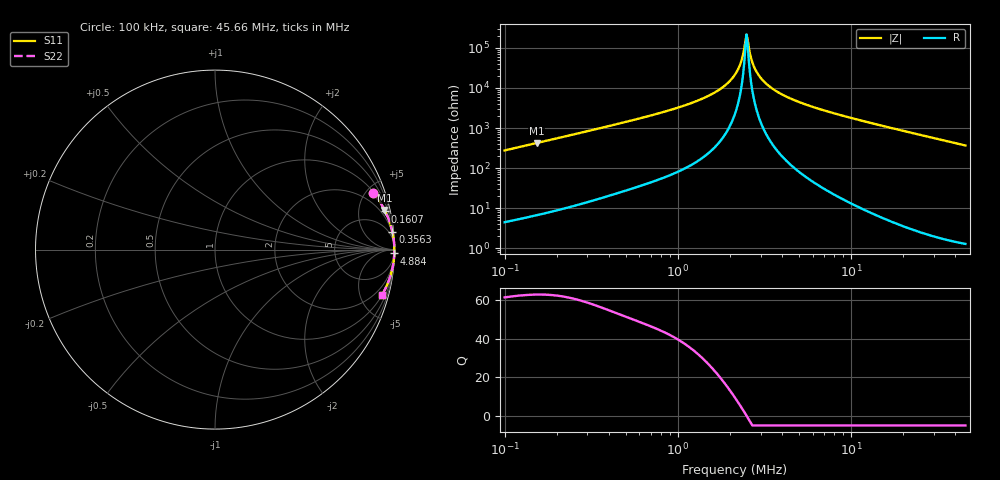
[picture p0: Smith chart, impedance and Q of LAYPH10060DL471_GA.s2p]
! LAYPH10060DL471_GA  S-PARAMETER MODEL  ( General Type )
! Model Generated by TAIYO YUDEN Corporation (http://www.ty-top.com)
! Version 3.0
! TAIYO YUDEN Control No. 180828NI43SB-FBB
! Copyright(c) 2017 TAIYO YUDEN CO.,LTD. All Rights Reserved.
! Product Description (link to TY-COMPAS)
! https://ds.yuden.co.jp/TYCOMPAS/or/detail?pn=LAYPH10060DL471MGA&u=M
! Products Name : Inductors
! Characteristics :
!  Inductance : 470 uH , SRF(min) : -Hz , DC Resistance(max) : 0.93 Ohm
!  Rated Current : Saturation :0.65 A , Temp Rise : 0.39 A (25 degC)
!  Case Size : 10.1 x 10.0 / 0.398 x 0.394 [mm/inch] , Thickness : 6 / 0.236 [mm/inch]
!  (Conditions: Temperature = 25 degC , DC Bias Current/Voltage = 0A / 0V)
! External Node Assignments :
!  1  o---GGG---o  2
! GND o---------o GND
! Frequency Range : 0.1MHz  -  45.660989MHz  [ 402 STEP ]
# MHz S RI R 50
! Freq[MHz].  S11 Real  S11 Imag  S21 Real  S21 Imag  S12 Real  S12 Imag  S22 Real  S22 Imag
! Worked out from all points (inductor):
!   401 points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, 100 kHz to 45.66 MHz, reference 50 ohm
!   read as one part in series: L = 439 uH near 103.1 kHz
!   highest Q = 63 at 153.5 kHz (marker M1), where L = 440 uH
!   self-resonance near 2.49 MHz
!   S11 on the Smith chart (normalised r, x): 100 kHz: 1.09, +5.54; 160.7 kHz: 1.14, +8.89; 356.3 kHz: 1, +20; 4.884 MHz: 3, -93; 45.66 MHz: 1.03, -7.37
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0.1  0.8808 0.316  0.1192 -0.316  0.1192 -0.316  0.8808 0.316
0.153521  0.9444 0.2214  0.0556 -0.2214  0.0556 -0.2214  0.9444 0.2214
0.160737  0.9488 0.2125  0.0512 -0.2125  0.0512 -0.2125  0.9488 0.2125
0.278916  0.9816 0.1263  0.0184 -0.1263  0.0184 -0.1263  0.9816 0.1263
0.356333  0.9883 0.099  0.0117 -0.099  0.0117 -0.099  0.9883 0.099
0.777943  0.9972 0.0425  0.00277 -0.0425  0.00277 -0.0425  0.9972 0.0425
1.158292  0.9987 0.0249  0.00132 -0.0249  0.00132 -0.0249  0.9987 0.0249
1.549339  0.9992 0.0146  0.000788 -0.0146  0.000788 -0.0146  0.9992 0.0146
1.890522  0.9994 0.00832  0.000585 -0.00832  0.000585 -0.00832  0.9994 0.00832
2.169809  0.9995 0.00414  0.000502 -0.00414  0.000502 -0.00414  0.9995 0.00414
2.306837  0.9995 0.00232  0.000479 -0.00232  0.000479 -0.00232  0.9995 0.00232
2.415258  0.9995 0.000952  0.000467 -0.000952  0.000467 -0.000952  0.9995 0.000952
2.490355  0.9995 4.37e-05  0.000462 -4.37e-05  0.000462 -4.37e-05  0.9995 4.37e-05
2.567787  0.9995 -0.000865  0.000458 0.000865  0.000458 0.000865  0.9995 -0.000865
2.647627  0.9995 -0.00177  0.000456 0.00177  0.000456 0.00177  0.9995 -0.00177
2.729949  0.9995 -0.00269  0.000456 0.00269  0.000456 0.00269  0.9995 -0.00269
3.038761  0.9995 -0.0059  0.000472 0.0059  0.000472 0.0059  0.9995 -0.0059
3.651597  0.9994 -0.0116  0.000556 0.0116  0.000556 0.0116  0.9994 -0.0116
4.884401  0.9991 -0.0215  0.000869 0.0215  0.000869 0.0215  0.9991 -0.0215
5.960003  0.9987 -0.0292  0.00126 0.0292  0.00126 0.0292  0.9987 -0.0292
16.62342  0.9903 -0.0959  0.00974 0.0959  0.00974 0.0959  0.9903 -0.0959
45.66099  0.9307 -0.2523  0.0693 0.2523  0.0693 0.2523  0.9307 -0.2523
